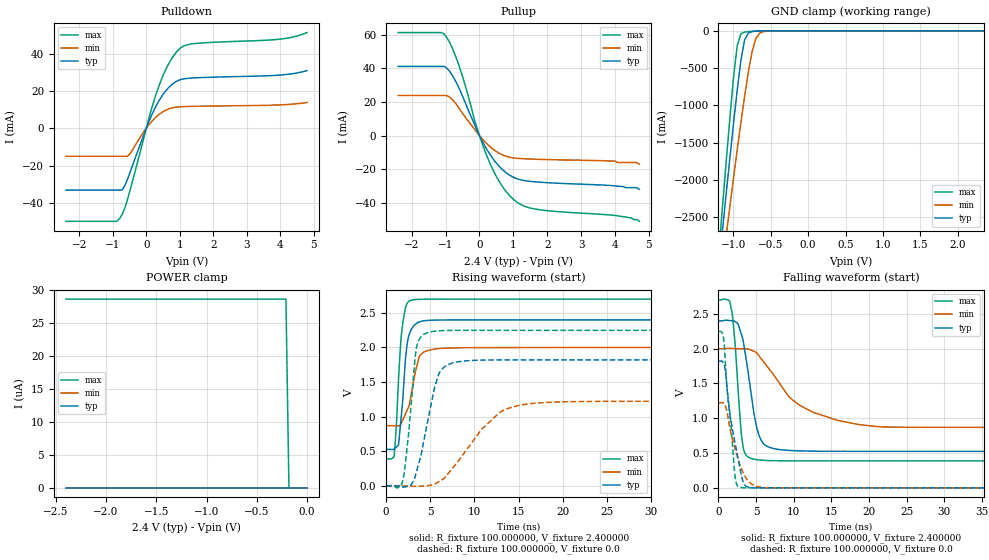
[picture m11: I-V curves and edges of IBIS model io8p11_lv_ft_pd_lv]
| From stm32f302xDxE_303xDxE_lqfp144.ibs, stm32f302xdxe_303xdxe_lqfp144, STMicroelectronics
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|   Model io8p11_lv_ft_pd_lv
[Model]  io8p11_lv_ft_pd_lv
Model_type I/O
Polarity   Non-Inverting
Enable   Active-Low
Vinl =   0.720000V
Vinh =   1.680000V
Vmeas =  1.200000V
Cref =   50.000000pF
Rref =   100.000000M
Vref =   0.0V
C_comp   5.024800pF   4.846300pF   5.260300pF
[Temperature Range]   25.000000   0.125000k   -40.000000
[Pullup Reference]   2.400000V   2.000000V   2.700000V
[Pulldown Reference]   0.0V   0.0V   0.0V
[POWER Clamp Reference]   2.400000V   2.000000V   2.700000V
[GND Clamp Reference]   0.0V   0.0V   0.0V
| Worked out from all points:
|   slope of the pulldown table from 0 to 0.36 V, typ, clamps not added: 25.5 ohm
|   slope of the pullup table from 0 to 0.36 V, typ, clamps not added: 28.4 ohm
|   GND clamp passes 1 mA (typ) near -0.60 V on its own axis
|   rising waveform, R_fixture 100.000000, V_fixture 2.400000: 20-80 % time 724ps typ, 1.17ns min, 637ps max; typ from 0.525 V to 2.4 V
|   rising waveform, R_fixture 100.000000, V_fixture 0.0: 20-80 % time 1.79ns typ, 4.7ns min, 953ps max; typ from 0 V to 1.82 V
|   falling waveform, R_fixture 100.000000, V_fixture 2.400000: 20-80 % time 1.6ns typ, 6.14ns min, 912ps max; typ from 2.4 V to 0.525 V
|   falling waveform, R_fixture 100.000000, V_fixture 0.0: 20-80 % time 1.58ns typ, 1.85ns min, 1.06ns max; typ from 1.82 V to 0 V
[Pulldown]
|Voltage   I(typ)   I(min)   I(max)
-2.4V     -33.16mA   -14.98mA   -49.86mA
-880mV    -33.16mA   -14.98mA   -49.86mA
-800mV    -33.16mA   -14.98mA   -48.55mA
-640mV    -30.75mA   -14.98mA   -42.77mA
-480mV    -23.43mA   -13.57mA   -32.92mA
80mV      3.651mA    1.905mA    5.506mA
400mV     15.37mA    7.665mA    23.73mA
720mV     22.75mA    10.69mA    36.23mA
1.04V     26.18mA    11.57mA    43.27mA
1.52V     27.09mA    11.81mA    45.55mA
4V        28.55mA    12.55mA    47.81mA
4.8V      30.9mA     13.81mA    51.31mA
[Pullup]
|Voltage   I(typ)   I(min)   I(max)
-2.4V     41.21mA    23.93mA    61.35mA
-1.12V    41.21mA    23.93mA    61.35mA
-960mV    40.07mA    23.79mA    58.27mA
-800mV    35.79mA    21.42mA    51.96mA
-560mV    26.32mA    15.02mA    38.93mA
-160mV    7.343mA    4.152mA    10.02mA
240mV     -8.976mA   -5.327mA   -13.21mA
640mV     -19.5mA    -11.09mA   -29.16mA
1.04V     -25.15mA   -13.38mA   -38.61mA
1.68V     -27.56mA   -14.07mA   -43.81mA
4V        -29.9mA    -15.2mA    -47.5mA
4.72V     -32mA      -17mA      -51mA
[GND_clamp]
|Voltage   I(typ)   I(min)   I(max)
-2.4V     -9.914A    -9.862A    -9.419A
-1.2V     -3.21A     -3.567A    -3.02A
-1.15V    -2.709A    -3.165A    -2.399A
-1.1V     -2.213A    -2.766A    -1.788A
-1.05V    -1.726A    -2.371A    -1.195A
-950mV    -800.5mA   -1.599A    -202.1mA
-900mV    -395mA     -1.228A    -38.18mA
-850mV    -120.2mA   -874.5mA   -15.93mA
-750mV    -9.822mA   -279.4mA   -7.289mA
-700mV    -4.75mA    -102mA     -4.527mA
-600mV    -1.046mA   -11.1mA    -938uA
2.35V     59.64uA    46.24uA    66.77uA
[POWER_clamp]
|Voltage   I(typ)   I(min)   I(max)
-2.4V     0A         0A         28.66uA
-210mV    0A         0A         28.66uA
-180mV    0A         0A         0A
0V        0A         0A         0A
[Ramp]
| variable   typ   min   max
dV/dt_r  1.09212/1.79278n   0.73260/4.70029n   1.34880/0.94894n
dV/dt_f  1.12442/1.60322n   0.67795/6.13687n   1.38698/0.91466n
R_load = 100.000000
[Rising Waveform]
R_fixture= 100.000000
V_fixture= 2.400000
V_fixture_min= 2.000000
V_fixture_max= 2.700000
|time   V(typ)   V(min)   V(max)
0s        524.8mV    868.7mV    387.2mV
900.9ps   530.7mV    867.7mV    416.8mV
1.401ns   591.1mV    866.2mV    1.541V
1.702ns   993mV      901.9mV    2.15V
2.002ns   1.483V     986.4mV    2.446V
2.402ns   2.071V     1.099V     2.645V
2.803ns   2.25V      1.296V     2.682V
3.804ns   2.372V     1.882V     2.696V
5.906ns   2.396V     1.982V     2.699V
49.85ns   2.399V     1.999V     2.699V
[Rising Waveform]
R_fixture= 100.000000
V_fixture= 0.0
V_fixture_min= 0.0
V_fixture_max= 0.0
|time   V(typ)   V(min)   V(max)
0s        -26.02uV   -10.95uV   -23.56uV
1.802ns   -20.37mV   -1.088mV   34.41mV
2.503ns   -8.357mV   -4.339mV   708.6mV
3.403ns   189mV      -9.857mV   1.973V
4.605ns   871.1mV    -1.209mV   2.21V
5.506ns   1.427V     24.13mV    2.235V
6.507ns   1.711V     99.83mV    2.244V
10.81ns   1.816V     817.5mV    2.248V
14.91ns   1.82V      1.159V     2.248V
49.85ns   1.82V      1.221V     2.248V
[Falling Waveform]
R_fixture= 100.000000
V_fixture= 2.400000
V_fixture_min= 2.000000
V_fixture_max= 2.700000
|time   V(typ)   V(min)   V(max)
0s        2.399V     1.999V     2.699V
1.301ns   2.406V     2.006V     2.7V
1.802ns   2.4V       2.004V     2.517V
3.103ns   2.184V     1.998V     717.8mV
4.104ns   1.534V     1.989V     433.1mV
5.405ns   749.2mV    1.893V     400.3mV
7.307ns   565.5mV    1.626V     390.5mV
10.81ns   531.1mV    1.185V     387.3mV
18.62ns   524.8mV    909.8mV    387.3mV
49.85ns   524.8mV    868.7mV    387.2mV
[Falling Waveform]
R_fixture= 100.000000
V_fixture= 0.0
V_fixture_min= 0.0
V_fixture_max= 0.0
|time   V(typ)   V(min)   V(max)
0s        1.82V      1.221V     2.248V
700.7ps   1.79V      1.215V     2.127V
1.101ns   1.484V     1.107V     1.478V
1.502ns   1.052V     859.2mV    1.079V
2.102ns   697.8mV    599.9mV    267.5mV
2.302ns   587.7mV    519.3mV    91.28mV
2.703ns   365.3mV    378.9mV    11.94mV
3.303ns   78.44mV    211.2mV    1.877mV
4.204ns   4.291mV    71.82mV    612.1uV
49.85ns   -26.02uV   -10.95uV   -23.56uV
